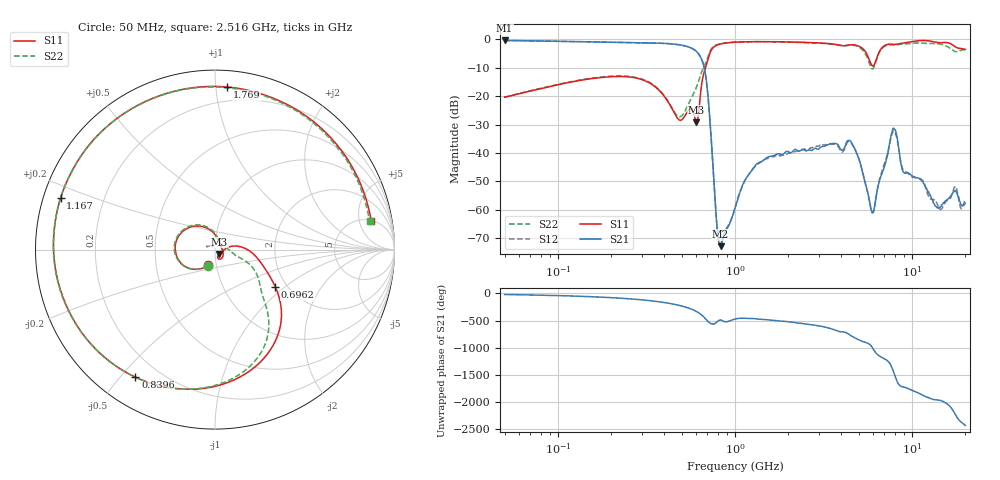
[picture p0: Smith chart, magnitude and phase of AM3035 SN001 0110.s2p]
# Hz S DB R 50
!freq MagS11 AngS11 MagS21 AngS21 MagS12 AngS12 MagS22 AngS22
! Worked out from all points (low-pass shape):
!   1601 points, 50 MHz to 20.05 GHz, reference 50 ohm
!   highest |S21| = -0.37 dB at 50 MHz (marker M1); lowest = -72.8 dB at 830.2 MHz (marker M2)
!   |S21| within 3 dB of the highest: start of sweep to 580.6 MHz
!   lowest |S11| = -29.2 dB at 606.1 MHz (marker M3), VSWR 1.07, Z = 52.5 - j2.52 ohm
!   |S11| at or under -10 dB: start of sweep to 681.7 MHz
!   |S22| runs from -27.3 to -0.8 dB; largest |S21 - S12| = 0.0041
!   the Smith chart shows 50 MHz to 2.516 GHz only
!   S11 on the Smith chart (normalised r, x): 50 MHz: 0.91, -0.16; 696.2 MHz: 1.74, -0.86; 839.6 MHz: 0.12, -0.55; 1.167 GHz: 0.05, +0.16; 1.769 GHz: 0.10, +1.07; 2.516 GHz: 5.16, +7.56
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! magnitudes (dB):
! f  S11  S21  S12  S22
! 50 MHz  -20.4  -0.4  -0.4  -20.3
! 135.9 MHz  -14.3  -0.8  -0.8  -14.2
! 369.6 MHz  -17.7  -1.3  -1.3  -17.5
! 487.7 MHz  -28.4  -1.9  -1.9  -27.3
! 606.1 MHz  -29.2  -4.2  -4.2  -16.9
! 696.2 MHz  -8.1  -16.6  -16.7  -7.1
! 790.8 MHz  -2.0  -65.5  -65.6  -1.9
! 830.2 MHz  -1.6  -72.8  -71.8  -1.5
! 839.6 MHz  -1.5  -72.1  -71.4  -1.5
! 1.005 GHz  -1.0  -59.2  -58.9  -1.0
! 1.167 GHz  -0.8  -48.6  -48.6  -0.8
! 1.769 GHz  -0.8  -40.3  -40.9  -0.9
! 2.516 GHz  -1.1  -39.3  -38.7  -1.2
! 2.722 GHz  -1.1  -39.1  -38.3  -1.2
! 4.497 GHz  -1.9  -35.8  -36.2  -2.0
! 6.001 GHz  -9.4  -61.0  -61.1  -10.4
! 7.402 GHz  -1.7  -38.2  -38.4  -1.9
! 7.978 GHz  -1.8  -31.7  -32.5  -2.0
! 8.994 GHz  -1.3  -46.8  -46.2  -1.6
! 14.37 GHz  -1.2  -59.1  -59.8  -1.6
! 17.45 GHz  -2.5  -53.4  -52.0  -4.2
! 20.05 GHz  -3.5  -57.7  -56.2  -3.6
